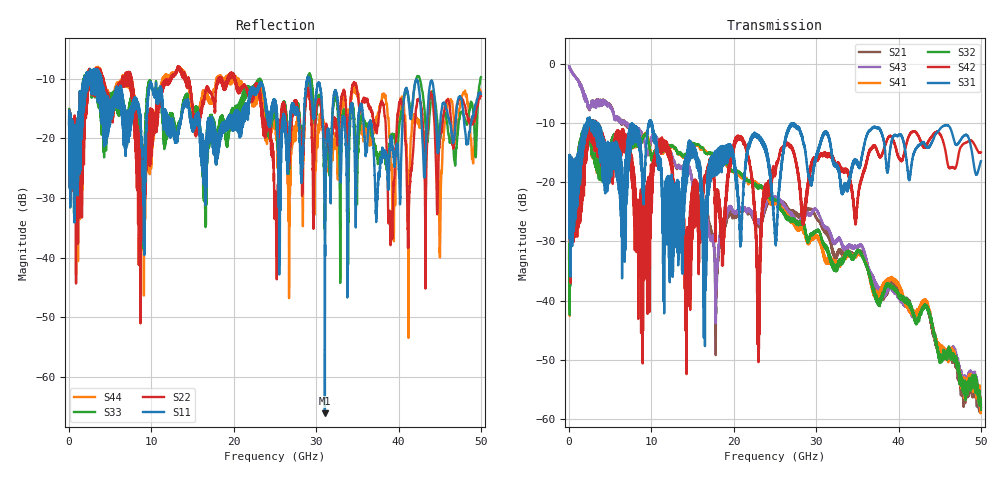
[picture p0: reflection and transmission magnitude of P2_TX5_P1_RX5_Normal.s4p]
!Keysight Technologies,N5225A,MY51441389,A.10.49.11
!Date: Monday, July 08, 2019 14:49:41
!Correction: S11(Full 4 Port(1,2,3,4))
!S12(Full 4 Port(1,2,3,4))
!S13(Full 4 Port(1,2,3,4))
!S14(Full 4 Port(1,2,3,4))
!S21(Full 4 Port(1,2,3,4))
!S22(Full 4 Port(1,2,3,4))
!S23(Full 4 Port(1,2,3,4))
!S24(Full 4 Port(1,2,3,4))
!S31(Full 4 Port(1,2,3,4))
!S32(Full 4 Port(1,2,3,4))
!S33(Full 4 Port(1,2,3,4))
!S34(Full 4 Port(1,2,3,4))
!S41(Full 4 Port(1,2,3,4))
!S42(Full 4 Port(1,2,3,4))
!S43(Full 4 Port(1,2,3,4))
!S44(Full 4 Port(1,2,3,4))
!S4P File: Measurements: <S11,S12,S13,S14>,
!<S21,S22,S23,S24>,
!<S31,S32,S33,S34>,
!<S41,S42,S43,S44>:
# Hz S  dB  R 50
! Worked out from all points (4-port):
!   5000 points, 10 MHz to 50 GHz, reference 50 ohm
!   strongest paths, dB at 10 MHz, 12.51 GHz, 25.01 GHz, 37.51 GHz, 50 GHz:
!     S31: -19.1, -22.4, -29.5, -10.9, -16.5
!     S42: -19.1, -16.7, -18.0, -15.2, -14.9
!     S32: -32.9, -13.8, -23.0, -39.8, -58.5
!     S41: -32.7, -13.9, -23.7, -38.8, -58.6
!     S43: -0.4, -15.7, -22.7, -37.6, -57.9
!     S21: -0.4, -15.7, -23.4, -38.5, -57.9
!   lowest |S11| = -66.1 dB at 31.06 GHz (marker M1), VSWR 1.00, Z = 50 + j0.029 ohm
!   |S11| at or under -10 dB: start of sweep to 1.836 GHz; 3.901 GHz to 28.92 GHz (25.01 GHz wide, 152 % of centre); 29.17 GHz to end of sweep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
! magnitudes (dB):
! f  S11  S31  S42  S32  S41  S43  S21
! 10 MHz  -17.8  -19.1  -19.1  -32.9  -32.7  -0.4  -0.4
! 2.21 GHz  -10.9  -10.4  -12.3  -11.2  -11.0  -6.6  -6.6
! 14.32 GHz  -14.8  -18.6  -40.5  -15.6  -15.8  -18.0  -17.9
! 20.9 GHz  -16.0  -30.0  -12.3  -18.7  -19.2  -24.6  -24.9
! 23.01 GHz  -11.4  -12.1  -43.1  -21.0  -20.7  -27.0  -27.5
! 31.06 GHz  -66.1  -11.9  -15.5  -30.5  -32.5  -27.4  -28.2
! 50 GHz  -12.5  -16.5  -14.9  -58.5  -58.6  -57.9  -57.9
